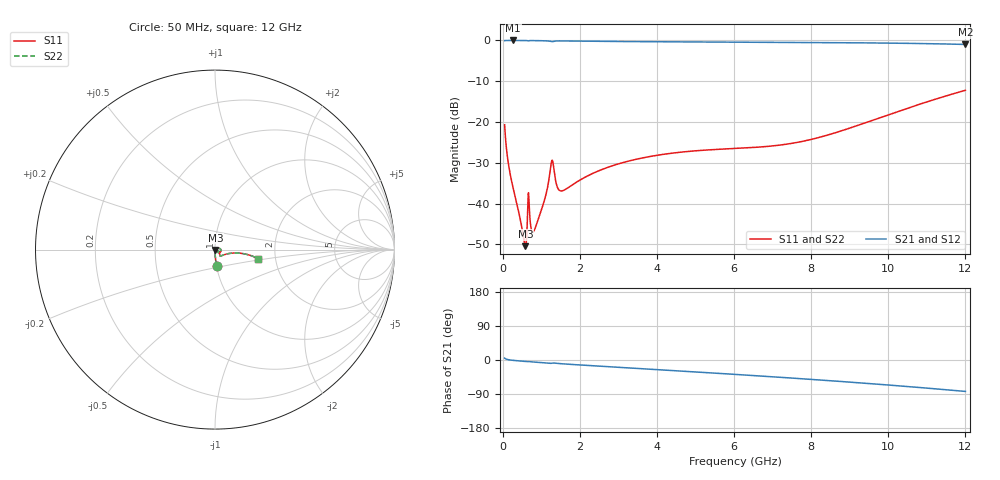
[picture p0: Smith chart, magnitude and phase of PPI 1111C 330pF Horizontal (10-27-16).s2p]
# MHz S MA R 50
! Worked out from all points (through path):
!   1601 points, 50 MHz to 12 GHz, reference 50 ohm
!   highest |S21| = -0.01 dB at 274.1 MHz (marker M1); lowest = -1.0 dB at 12 GHz (marker M2)
!   group delay of S21, straight-line fit = 18.7 ps
!   lowest |S11| = -50.4 dB at 587.8 MHz (marker M3), VSWR 1.01, Z = 50.3 - j0.163 ohm
!   |S11| at or under -10 dB: start of sweep to end of sweep
!   |S22| runs from -50.4 to -12.2 dB; largest |S21 - S12| = 0
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50  0.09257 -84.6  0.995 5.0  0.995 5.0  0.09257 -84.6
162.0312  0.02806 -88.4  0.9991 0.5  0.9991 0.5  0.02806 -88.4
274.0625  0.01531 -89.3  0.9994 -1.0  0.9994 -1.0  0.01531 -89.3
542.9375  0.003793 -62.6  0.998 -3.4  0.998 -3.4  0.003793 -62.6
587.75  0.003009 -32.5  0.9973 -3.8  0.9973 -3.8  0.003009 -32.5
640.0312  0.006309 16.1  0.994 -4.4  0.994 -4.4  0.006309 16.1
684.8438  0.01008 -48.9  0.9928 -4.2  0.9928 -4.2  0.01008 -48.9
707.25  0.006585 -51.8  0.9955 -4.4  0.9955 -4.4  0.006585 -51.8
774.4688  0.004474 -25.0  0.9957 -5.1  0.9957 -5.1  0.004474 -25.0
871.5625  0.005461 2.6  0.9945 -5.9  0.9945 -5.9  0.005461 2.6
1095.625  0.01155 22.3  0.9899 -7.6  0.9899 -7.6  0.01155 22.3
1274.875  0.03375 -7.4  0.9662 -8.5  0.9662 -8.5  0.03375 -7.4
1319.688  0.02834 -37.0  0.975 -8.0  0.975 -8.0  0.02834 -37.0
1416.781  0.01596 -40.9  0.9863 -8.9  0.9863 -8.9  0.01596 -40.9
1498.938  0.01433 -32.3  0.9867 -9.7  0.9867 -9.7  0.01433 -32.3
2044.156  0.01992 -24.0  0.9803 -13.3  0.9803 -13.3  0.01992 -24.0
2918  0.02986 -36.2  0.9713 -18.7  0.9713 -18.7  0.02986 -36.2
4038.312  0.03935 -47.7  0.9632 -25.5  0.9632 -25.5  0.03935 -47.7
6025  0.04742 -49.9  0.9532 -37.9  0.9532 -37.9  0.04742 -49.9
8019.156  0.06148 -26.4  0.9435 -51.3  0.9435 -51.3  0.06148 -26.4
10013.31  0.1232 -8.8  0.9275 -66.1  0.9275 -66.1  0.1232 -8.8
12000  0.2451 -11.8  0.893 -82.9  0.893 -82.9  0.2451 -11.8
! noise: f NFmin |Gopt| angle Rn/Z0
50  0.000587  0.9129  0.3557  0.001485
1372  0.01416  0.9021  9.132  0.03149
2701  0.02591  0.8966  17.85  0.05341
4031  0.03676  0.8942  26.35  0.07187
5360  0.04561  0.8907  34.54  0.0829
6682  0.05343  0.8886  42.33  0.09077
8012  0.06086  0.8884  49.75  0.09762
9341  0.06823  0.8898  56.74  0.1044
1.067e+04  0.0758  0.8929  63.29  0.1119
1.2e+04  0.08379  0.8971  69.41  0.1204
